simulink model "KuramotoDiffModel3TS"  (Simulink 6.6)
settings: Solver=ode3  StartTime=0.0  StopTime=Tend  FixedStep=dt  RelTol=1e-8
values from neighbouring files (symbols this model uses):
  k = k+1    (= 1)    [charPathLength.m]    (also in SyncKuramotoDemo.m = 0.2)
  omega = 1    [ConvergenceDemo.m]    (also in PlatoonDemo.m = 0.7; SyncIMPDemo.m = 3; SyncKuramotoDemo.m = [0.4)
  x0 = x0/sum(x0)*N1    [ConsensusDemo.m]    (also in EventtriggeredPendulum.m = [0; 0.18; 0; 0]; LCLCNetworkDemo.m = [x01; zeros((N1-1)*n, 1)]; LCNetworkDemo.m = [1 0 0.5 0 -1 0]; NetwPendulum.m = [0; 0; 0.05; 0])

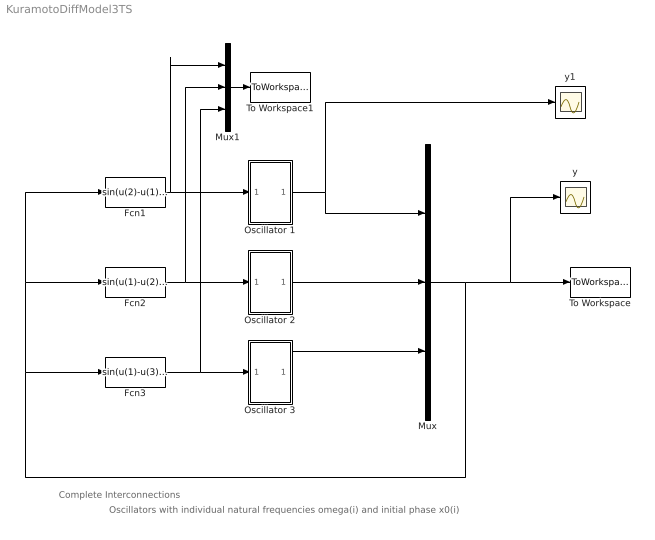
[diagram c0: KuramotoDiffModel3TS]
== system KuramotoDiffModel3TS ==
  note: Oscillators with individual natural frequencies omega(i) and initial phase x0(i)
  note: Complete Interconnections
  Fcn1 : Fcn  Expr=sin(u(2)-u(1))+sin(u(3)-u(1))
  Fcn2 : Fcn  Expr=sin(u(1)-u(2))+sin(u(3)-u(2))
  Fcn3 : Fcn  Expr=sin(u(1)-u(3))+sin(u(2)-u(3))
  Mux : Mux  Inputs=3
  Mux1 : Mux  Inputs=3
  Oscillator 1 : Subsystem
  Oscillator 2 : Subsystem
  Oscillator 3 : Subsystem
  To Workspace : ToWorkspace  VariableName=Theta  SampleTime=-1  SaveFormat=Array
  To Workspace1 : ToWorkspace  VariableName=e  SampleTime=-1  SaveFormat=Array
  y : Scope
  y1 : Scope
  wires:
  Oscillator 1/1(Out1) -> Mux/1, y1/1
  Oscillator 3/1(Out1) -> Mux/3
  Mux/1 -> To Workspace/1, y/1, Fcn1/1, Fcn2/1, Fcn3/1
  Fcn1/1 -> Oscillator 1/1(In1), Mux1/1
  Fcn2/1 -> Oscillator 2/1(In1), Mux1/2
  Fcn3/1 -> Oscillator 3/1(In1), Mux1/3
  Oscillator 2/1(Out1) -> Mux/2
  Mux1/1 -> To Workspace1/1

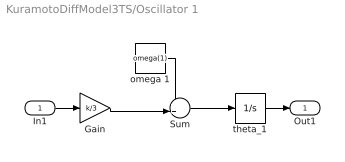
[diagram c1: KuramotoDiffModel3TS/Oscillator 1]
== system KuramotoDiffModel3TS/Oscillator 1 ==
  In1 : Inport
  Gain : Gain  Gain=k/3
  Sum : Sum  Inputs=++|
  omega 1 : Constant  Value=omega(1)
  theta_1 : Integrator  InitialCondition=x0(1)
  Out1 : Outport
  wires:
  omega 1/1 -> Sum/1
  Gain/1 -> Sum/2
  Sum/1 -> theta_1/1
  In1/1 -> Gain/1
  theta_1/1 -> Out1/1

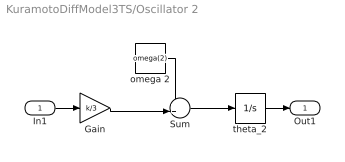
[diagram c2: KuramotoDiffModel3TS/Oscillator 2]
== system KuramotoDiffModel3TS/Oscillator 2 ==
  In1 : Inport
  Gain : Gain  Gain=k/3
  Sum : Sum  Inputs=++|
  omega 2 : Constant  Value=omega(2)
  theta_2 : Integrator  InitialCondition=x0(2)
  Out1 : Outport
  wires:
  omega 2/1 -> Sum/1
  Gain/1 -> Sum/2
  Sum/1 -> theta_2/1
  In1/1 -> Gain/1
  theta_2/1 -> Out1/1

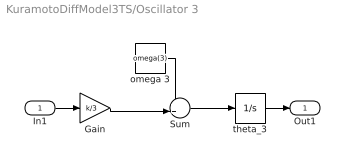
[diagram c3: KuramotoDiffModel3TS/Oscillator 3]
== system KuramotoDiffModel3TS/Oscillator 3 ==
  In1 : Inport
  Gain : Gain  Gain=k/3
  Sum : Sum  Inputs=++|
  omega 3 : Constant  Value=omega(3)
  theta_3 : Integrator  InitialCondition=x0(3)
  Out1 : Outport
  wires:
  omega 3/1 -> Sum/1
  Gain/1 -> Sum/2
  Sum/1 -> theta_3/1
  In1/1 -> Gain/1
  theta_3/1 -> Out1/1
